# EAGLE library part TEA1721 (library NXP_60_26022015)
HV start-up flyback controller with integrated MOSFET for 5 W applications The TEA1721 is a small and low cost module Switched Mode Power Supply (SMPS) controller IC for low power applications (up to 5 W) and operates directly from the rectified universal mains input. The device includes a high voltage power switch (700 V) and has been optimized for flyback converter topologies to provide high-efficiency over the entire load range with ultra-low power consumption in the no-load condition. It provides a circuit for start-up directly from the rectified mains voltage without any external bleeder circuits. The converter operates as a regulated voltage source from no-load up to the maximum output current and operates as current source that delivers the maximum current over a broad output voltage range. Using the TEA1721, a low power converter can be built at minimum cost and with the minimum number of external components. The controller regulates the output voltage with primary-side sensing which eliminates the need for an additional secondary feedback circuitry and simplifies the design. At higher power levels, a frequency and current control mode is used. It operates with Burst mode control at low power levels and no-load condition. The burst mode minimizes audible noise and provides an energy saver state which reduces the power consumption in no-load condition. AAL Eindhoven MK
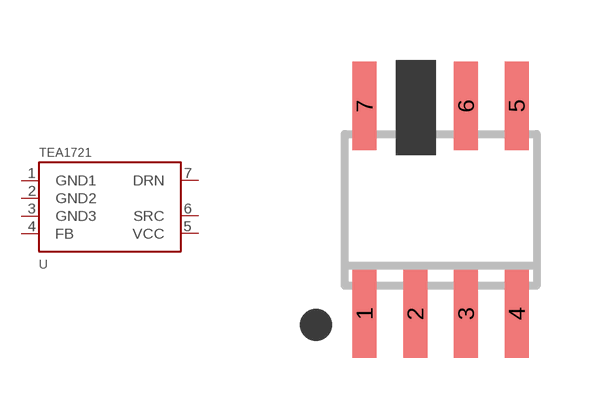
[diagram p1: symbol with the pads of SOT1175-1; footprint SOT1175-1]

Designator prefix U

## TEA1721AT (12NC: 9352 968 88118; BURST: 430 Hz), TEA1721BT (12NC: 9352 968 94118; BURST: 905 Hz), TEA1721DT (12NC: 9352 968 89118; BURST: 1270 Hz), TEA1721FT (12NC: 9352 968 87118; BURST: 1750 Hz)  [SOT1175-1]
1  GND1  pwr
2  GND2  pwr
3  GND3  pwr
4  FB
5  VCC  pwr
6  SRC  in
7  DRN  out

## Footprint SOT1175-1 (pad centres in mm)
SOT1175-1 SO7: plastic small outline package; 7 leads; body width 3.9 m JEDEC: --- IEC: ---
smd 0.6 x 2.2: 1 -1.905,-2.6; 2 -0.635,-2.6; 3 0.635,-2.6; 4 1.905,-2.6; 5 1.905,2.6; 6 0.635,2.6; 7 -1.905,2.6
